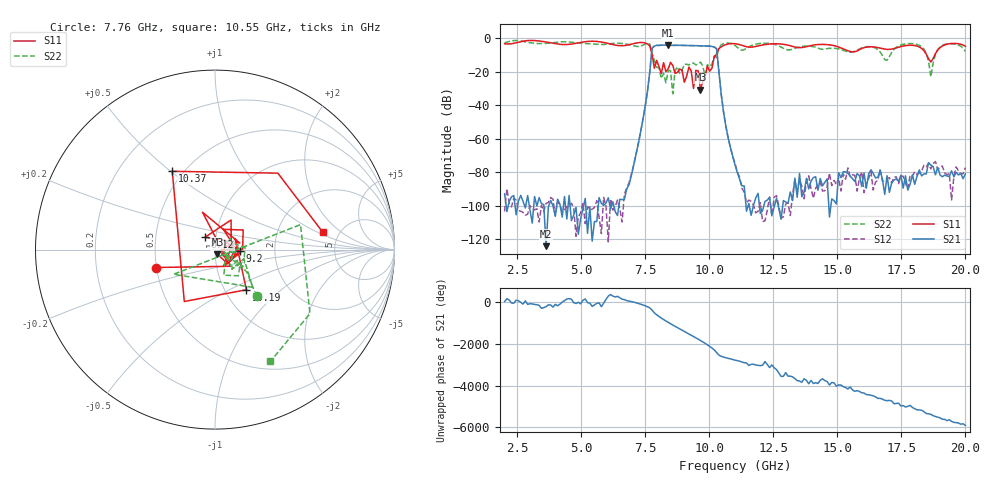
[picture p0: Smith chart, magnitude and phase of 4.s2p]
!Keysight Technologies,N5234A,MY52241180,A.10.60.03
!Date: Friday, January 20, 2023 09:33:24
!Correction: S11(Full 2 Port(1,2))
!S21(Full 2 Port(1,2))
!S12(Full 2 Port(1,2))
!S22(Full 2 Port(1,2))
!S2P File: Measurements: S11, S21, S12, S22:
# Hz S  dB  R 50
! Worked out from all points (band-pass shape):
!   201 points, 2 GHz to 20 GHz, reference 50 ohm
!   highest |S21| = -4.07 dB at 8.39 GHz (marker M1); lowest = -124.2 dB at 3.62 GHz (marker M2)
!   |S21| within 3 dB of the highest: 7.753 GHz to 10.29 GHz (2.533 GHz wide, 28.1 % of centre)
!   lowest |S11| = -30.6 dB at 9.65 GHz (marker M3), VSWR 1.06, Z = 51.3 - j2.68 ohm
!   |S11| at or under -10 dB: 7.768 GHz to 10.25 GHz (2.48 GHz wide, 27.5 % of centre); 18.49 GHz to 18.8 GHz (315.6 MHz wide, 1.69 % of centre)
!   |S22| runs from -33.1 to -1.3 dB; largest |S21 - S12| = 0.00041
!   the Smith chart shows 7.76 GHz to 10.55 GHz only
!   S11 on the Smith chart (normalised r, x): 7.76 GHz: 0.50, -0.11; 8.12 GHz: 0.89, +0.12; 9.2 GHz: 1.32, -0.01; 10.19 GHz: 1.26, -0.61; 10.37 GHz: 0.44, +0.51; 10.55 GHz: 3.73, +1.14
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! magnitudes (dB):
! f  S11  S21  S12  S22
! 2 GHz  -3.3  -92.9  -103.4  -2.7
! 3.62 GHz  -2.2  -124.2  -98.6  -3.0
! 5.06 GHz  -2.2  -101.8  -98.3  -3.0
! 6.95 GHz  -3.5  -82.1  -81.1  -4.1
! 7.76 GHz  -9.3  -6.0  -6.0  -9.1
! 8.03 GHz  -16.9  -4.3  -4.3  -17.5
! 8.12 GHz  -21.1  -4.1  -4.1  -23.9
! 8.39 GHz  -18.3  -4.1  -4.1  -19.4
! 8.57 GHz  -16.2  -4.2  -4.2  -33.1
! 8.66 GHz  -20.9  -4.2  -4.2  -19.2
! 9.2 GHz  -17.2  -4.3  -4.3  -15.9
! 9.65 GHz  -30.6  -4.5  -4.5  -14.2
! 10.19 GHz  -10.9  -5.2  -5.2  -10.5
! 10.37 GHz  -6.1  -19.6  -19.6  -6.1
! 10.55 GHz  -4.3  -43.8  -43.8  -3.2
! 11 GHz  -3.2  -75.6  -74.6  -4.2
! 14.06 GHz  -4.0  -83.2  -95.5  -5.0
! 17.03 GHz  -6.6  -92.0  -83.3  -10.9
! 18.2 GHz  -5.2  -78.6  -80.5  -4.2
! 18.65 GHz  -14.1  -75.7  -78.0  -23.0
! 19.01 GHz  -5.6  -81.7  -77.1  -5.2
! 20 GHz  -4.8  -81.0  -77.2  -7.8
